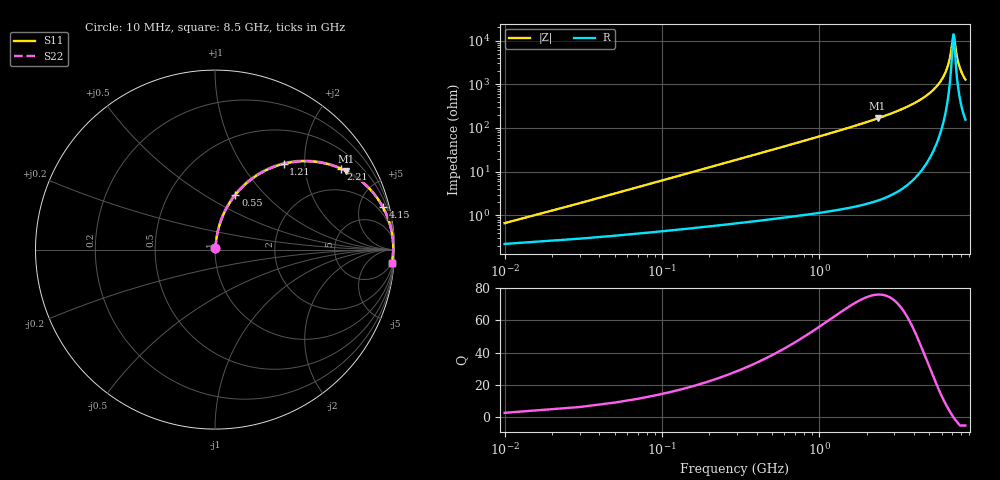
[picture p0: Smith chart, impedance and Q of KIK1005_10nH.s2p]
!version-3
!date-01.2023
!Series
# MHz S RI R 50
!Freq ReS11 ImS11 ReS21 ImS21 ReS12 ImS12 ReS22 ImS22
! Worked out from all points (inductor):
!   426 points, 10 MHz to 8.5 GHz, reference 50 ohm
!   read as one part in series: L = 10 nH near 50 MHz
!   highest Q = 76 at 2.35 GHz (marker M1), where L = 11.2 nH
!   self-resonance near 7.13 GHz
!   S11 on the Smith chart (normalised r, x): 10 MHz: 1.00, +0.01; 550 MHz: 1.02, +0.70; 1.21 GHz: 1.03, +1.57; 2.21 GHz: 1.04, +3.07; 4.15 GHz: 1.15, +7.87; 8.5 GHz: 4, -25
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10  0.00227 0.00625  0.9977 -0.00625  0.9977 -0.00625  0.00227 0.00625
70  0.00573 0.0436  0.9943 -0.0436  0.9943 -0.0436  0.00573 0.0436
90  0.00731 0.0559  0.9927 -0.0559  0.9927 -0.0559  0.00731 0.0559
170  0.0164 0.1046  0.9836 -0.1046  0.9836 -0.1046  0.0164 0.1046
330  0.0474 0.1966  0.9526 -0.1966  0.9526 -0.1966  0.0474 0.1966
550  0.1138 0.3055  0.8862 -0.3055  0.8862 -0.3055  0.1138 0.3055
1210  0.3818 0.4778  0.6182 -0.4778  0.6182 -0.4778  0.3818 0.4778
1430  0.4675 0.4915  0.5325 -0.4915  0.5325 -0.4915  0.4675 0.4915
2210  0.6998 0.4518  0.3002 -0.4518  0.3002 -0.4518  0.6998 0.4518
2350  0.73 0.4374  0.27 -0.4374  0.27 -0.4374  0.73 0.4374
2850  0.816 0.3808  0.184 -0.3808  0.184 -0.3808  0.816 0.3808
4150  0.9352 0.2365  0.0648 -0.2365  0.0648 -0.2365  0.9352 0.2365
4270  0.9415 0.2245  0.0585 -0.2245  0.0585 -0.2245  0.9415 0.2245
5670  0.9839 0.1018  0.0161 -0.1018  0.0161 -0.1018  0.9839 0.1018
6210  0.9901 0.0618  0.00992 -0.0618  0.00992 -0.0618  0.9901 0.0618
6590  0.9922 0.0357  0.00776 -0.0357  0.00776 -0.0357  0.9922 0.0357
6850  0.9929 0.0187  0.00715 -0.0187  0.00715 -0.0187  0.9929 0.0187
7090  0.9929 0.00362  0.00712 -0.00362  0.00712 -0.00362  0.9929 0.00362
7190  0.9927 -0.00253  0.00725 0.00253  0.00725 0.00253  0.9927 -0.00253
7450  0.9921 -0.0181  0.00795 0.0181  0.00795 0.0181  0.9921 -0.0181
7730  0.9908 -0.0342  0.00922 0.0342  0.00922 0.0342  0.9908 -0.0342
8500  0.9849 -0.0755  0.0151 0.0755  0.0151 0.0755  0.9849 -0.0755
